{attribute 'Tc2GvlVarNames'}
(*配方功能: 第三方触摸屏*)

VAR_GLOBAL CONSTANT
	MAX_FILE_NAME_STR			: INT	:= 20;	(*配方名字长度, 20个字节*)
	MAX_RECIPE_FILES			: INT	:= 5;	(*最多保存的配方数量*)
END_VAR

VAR_GLOBAL
(*配方文件(和配方号对应的)名字*)
	H_RecipeName				: ARRAY[0..MAX_RECIPE_FILES] OF STRING(MAX_FILE_NAME_STR);
END_VAR

VAR_GLOBAL
	H_CurRecipeNum				: INT;	(*当前配方号*)
	H_SetRecipeNum				: INT;	(*设定配方号, 0~100*)
(*!!!按钮, 下降沿触发!!!*)
	H_RecipeLoad				: BOOL;	(*读取设定配方号中的参数*)
	H_RecipeSave				: BOOL;	(*参数保存到当前配方号*)
	H_RecipeSaveAs				: BOOL;	(*参数保存到设定的配方号*)
(*状态*)
	H_RecipeInitialDone			: BOOL;	(*初始化完成*)
	H_RecipeDone				: BOOL;	(*读写完成*)
	H_RecipeBusy				: BOOL;	(*读写中*)
	H_RecipeError				: BOOL;	(*读写失败*)
	H_RecipeLoading				: BOOL;	(*配方读取中...*)
	H_RecipeSaving				: BOOL;	(*配方保存中...*)
	H_NewRecipeSaving			: BOOL;	(*配方另存中...*)
	H_CurDataAutoSaving			: BOOL;	(*自动保存中...*)
(*当前配方名*)
	H_CurRecName				: STRING(MAX_FILE_NAME_STR);
END_VAR
